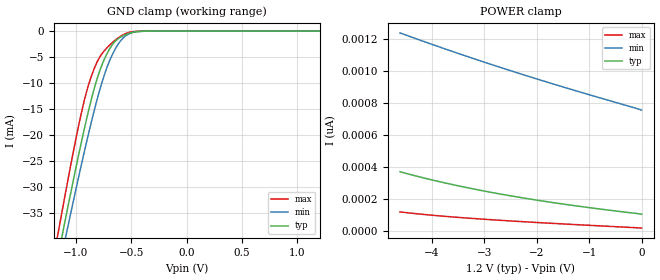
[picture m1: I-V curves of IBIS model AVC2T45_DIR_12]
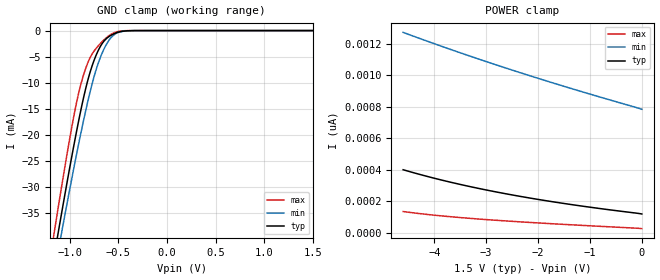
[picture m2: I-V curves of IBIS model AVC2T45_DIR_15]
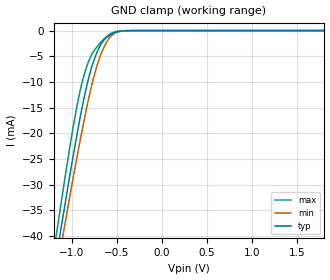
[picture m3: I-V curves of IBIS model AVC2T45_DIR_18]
| TEXAS INSTRUMENTS INCORPORATED
| Standard Linear and Logic Group
| IBIS Model of SN74AVC2T45
| DUAL-BIT DUAL-SUPPLY BUS TRANSCEIVER WITH CONFIGURABLE VOLTAGE
| TRANSLATION AND 3-STATE OUTPUTS
| This file contains package information for the following:
|  SOT 8-pin (DCT) package as [Component] AVC2T45_DCT
|  SOT 8-pin (DCU) package as [Component] AVC2T45_DCU
|  NanoStar WCSP 8-pin (YEP) package as [Component] AVC2T45_YEP
|  NanoFree WCSP 8-pin (YZP) package as [Component] AVC2T45_YZP
|  NanoFree WCSP 8-pin (YZT) package as [Component] AVC2T45_YZT
| This device can be powered at the following Vccs:
|  1.2 volt Vcc
|  1.5 volt Vcc
|  1.8 volt Vcc
|  2.5 volt Vcc
|  3.3 volt Vcc
| This file provides unique models under the [Model Selector] for each Vcc.
| For operation at a specific Vcc, select the appropriate model after each
| [Model Selector] keyword.
[IBIS Ver]   3.2
[Comment char]  |_char
[File Name]   sn74avc2t45.ibs
[File Rev]   1.2 | x_die
[Date]   February 22, 2005
[Source]   Data created from TI-SPICE simulations at TI-SLL.
[Notes]   The following is an IBIS list for the AVC2T45.
   Please contact sllibis@ti.com with questions and
   comments concerning SLL IBIS models.
   - 1.1 Release IBIS file on 04/23/04
   - 1.2 YEP, YZP, and YZT packages added. 02/22/05
   - Power clamp data deleted as there is no power-clamp diode.
   - Due to the fact that the Device is 4.6-V Input/Output
   tolarent, the I/O models has some Non-Monotonic Warnings.
   - End point warning due to AC and DC mismatch.
[Disclaimer] Property of Texas Instruments Incorporated.  Unauthorized
   reproduction and/or distribution is strictly prohibited.
   This product is protected under copyright law.
   Created  2004, (C) Copyright  2004, Texas Instruments
   Incorporated, All Rights Reserved
   UNLESS THERE IS A SIGNED, WRITTEN AGREEMENT TO THE
   CONTRARY, TEXAS INSTRUMENTS (TI) IS PROVIDING THE IBIS
   MODELS  AND WITHOUT ANY WARRANTY, EXPRESSED OR
   IMPLIED.  TI assumes no liability for:
   1) the accuracy of the IBIS models provided to your
   company;
   2) the proper functioning of these IBIS Models in your
   design or for any resulting applications; or
   3) infringement of patents, copyrights or intellectual
   property rights resulting from your use of these IBIS
   models.
   TI provides IBIS Models as a service to our customers.
   You and your company shall not distribute, sell or give
   these models to anyone else without prior written
   permission from TI.
   TI reserves the right to make changes to our products or
   to discontinue any semiconductor product or service
   without notice, and advises our customers to obtain the
   latest version of relevant information to verify, before
   placing orders, that the information being relied on is
   current.
   Please be aware that your receipt and use of the IBIS
   information provided shall serve as acceptance of these
   terms and conditions.  If you do not accept these terms,
   you should return or destroy the IBIS models and any
   other accompanying information immediately.
| Component AVC2T45_DCT 8-pin SOT
[Component]   AVC2T45_DCT
[Manufacturer]   Texas Instruments, Inc.
[Package]
|   typ   min   max
R_pkg   2.900e-02   2.800e-02   3.100e-02
L_pkg   1.796e-09   1.666e-09   1.924e-09
C_pkg   2.310e-13   2.210e-13   2.420e-13
[Pin]   signal_name   model_name   R_pin   L_pin   C_pin
1   VCCA   POWER   3.100e-02   1.894e-09   2.230e-13
2   A1   AVC2T45_IOA   2.800e-02   1.697e-09   2.370e-13
3   A2   AVC2T45_IOA   3.000e-02   1.722e-09   2.390e-13
4   GND   GND   3.000e-02   1.861e-09   2.210e-13
5   DIR   AVC2T45_DIR   2.800e-02   1.924e-09   2.280e-13
6   B2   AVC2T45_IOB   2.900e-02   1.736e-09   2.420e-13
7   B1   AVC2T45_IOB   2.800e-02   1.666e-09   2.360e-13
8   VCCB   POWER   3.000e-02   1.871e-09   2.220e-13
| Component AVC2T45_DCU 8-pin SOT
[Component]   AVC2T45_DCU
[Manufacturer]   Texas Instruments, Inc.
[Package]
|   typ   min   max
R_pkg   2.600e-02   2.300e-02   3.800e-02
L_pkg   1.394e-09   1.066e-09   2.046e-09
C_pkg   2.590e-13   2.150e-13   3.720e-13
[Pin]   signal_name   model_name   R_pin   L_pin   C_pin
1   VCCA   POWER   2.400e-02   1.520e-09   2.710e-13
2   A1   AVC2T45_IOA   2.300e-02   1.112e-09   2.180e-13
3   A2   AVC2T45_IOA   2.300e-02   1.070e-09   2.170e-13
4   GND   GND   2.700e-02   2.046e-09   3.720e-13
5   DIR   AVC2T45_DIR   2.700e-02   1.542e-09   2.730e-13
6   B2   AVC2T45_IOB   2.300e-02   1.100e-09   2.240e-13
7   B1   AVC2T45_IOB   2.300e-02   1.066e-09   2.150e-13
8   VCCB   POWER   3.800e-02   1.696e-09   2.800e-13
| Component AVC2T45_YEP 8-pin NanoStar WCSP
[Component]   AVC2T45_YEP
[Manufacturer]   Texas Instruments, Inc.
[Package]
|   typ   min   max
R_pkg   0.001   0.001   0.001
L_pkg   0.021nH   0.021nH   0.021nH
C_pkg   0.043pF   0.042pF   0.044pF
[Pin]   signal_name   model_name   R_pin   L_pin   C_pin
1   VCCA   POWER   0.046   2.861nH   0.321pF
2   A1   AVC2T45_IOA   0.037   2.437nH   0.286pF
3   A2   AVC2T45_IOA   0.034   2.419nH   0.286pF
4   GND   GND   0.043   2.784nH   0.321pF
5   DIR   AVC2T45_DIR   0.043   2.784nH   0.321pF
6   B2   AVC2T45_IOB   0.035   2.420nH   0.286pF
7   B1   AVC2T45_IOB   0.037   2.437nH   0.286pF
8   VCCB   POWER   0.046   2.860nH   0.321pF
| Component AVC2T45_YZP 8-pin NanoFree WCSP
[Component]   AVC2T45_YZP
[Manufacturer]   Texas Instruments, Inc.
[Package]
|   typ   min   max
R_pkg   0.001   0.001   0.001
L_pkg   0.021nH   0.021nH   0.021nH
C_pkg   0.043pF   0.042pF   0.044pF
[Pin]   signal_name   model_name   R_pin   L_pin   C_pin
1   VCCA   POWER   0.046   2.861nH   0.321pF
2   A1   AVC2T45_IOA   0.037   2.437nH   0.286pF
3   A2   AVC2T45_IOA   0.034   2.419nH   0.286pF
4   GND   GND   0.043   2.784nH   0.321pF
5   DIR   AVC2T45_DIR   0.043   2.784nH   0.321pF
6   B2   AVC2T45_IOB   0.035   2.420nH   0.286pF
7   B1   AVC2T45_IOB   0.037   2.437nH   0.286pF
8   VCCB   POWER   0.046   2.860nH   0.321pF
| Component AVC2T45_YZT 8-pin NanoFree WCSP
[Component]   AVC2T45_YZT
[Manufacturer]   Texas Instruments, Inc.
[Package]
|   typ   min   max
R_pkg   0.001   0.001   0.001
L_pkg   0.021nH   0.021nH   0.021nH
C_pkg   0.043pF   0.042pF   0.044pF
[Pin]   signal_name   model_name   R_pin   L_pin   C_pin
1   VCCA   POWER   0.046   2.861nH   0.321pF
2   A1   AVC2T45_IOA   0.037   2.437nH   0.286pF
3   A2   AVC2T45_IOA   0.034   2.419nH   0.286pF
4   GND   GND   0.043   2.784nH   0.321pF
5   DIR   AVC2T45_DIR   0.043   2.784nH   0.321pF
6   B2   AVC2T45_IOB   0.035   2.420nH   0.286pF
7   B1   AVC2T45_IOB   0.037   2.437nH   0.286pF
8   VCCB   POWER   0.046   2.860nH   0.321pF
| Model AVC2T45_DIR
[Model Selector]   AVC2T45_DIR
AVC2T45_DIR_12   1.2 volt Vcc
AVC2T45_DIR_15   1.5 volt Vcc
AVC2T45_DIR_18   1.8 volt Vcc
AVC2T45_DIR_25   2.5 volt Vcc
AVC2T45_DIR_33   3.3 volt Vcc
| Model AVC2T45_IOA
[Model Selector]   AVC2T45_IOA
AVC2T45_IOA_12   1.2 volt Vcc
AVC2T45_IOA_15   1.5 volt Vcc
AVC2T45_IOA_18   1.8 volt Vcc
AVC2T45_IOA_25   2.5 volt Vcc
AVC2T45_IOA_33   3.3 volt Vcc
| Model AVC2T45_IOB
[Model Selector]   AVC2T45_IOB
AVC2T45_IOB_12   1.2 volt Vcc
AVC2T45_IOB_15   1.5 volt Vcc
AVC2T45_IOB_18   1.8 volt Vcc
AVC2T45_IOB_25   2.5 volt Vcc
AVC2T45_IOB_33   3.3 volt Vcc
| Models and submodels in the file (15): AVC2T45_DIR_12 (Input), AVC2T45_DIR_15 (Input), AVC2T45_DIR_18 (Input), AVC2T45_DIR_25 (Input), AVC2T45_DIR_33 (Input), AVC2T45_IOA_12 (I/O), AVC2T45_IOA_15 (I/O), AVC2T45_IOA_18 (I/O), AVC2T45_IOA_25 (I/O), AVC2T45_IOA_33 (I/O), AVC2T45_IOB_12 (I/O), AVC2T45_IOB_15 (I/O), AVC2T45_IOB_18 (I/O), AVC2T45_IOB_25 (I/O), AVC2T45_IOB_33 (I/O)
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[Model]   AVC2T45_DIR_12
Model_type  Input
Vinl=0.42
Vinh=0.78
| variable   typ   min   max
C_comp   2.46pF   2.11pF   2.89pF
[Temperature Range]   40   100   -40
| Ambient temperature   25   85   -40
[Voltage range]   1.2   NA   NA
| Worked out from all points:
|   GND clamp passes 1 mA (typ) near -0.58 V on its own axis
[GND Clamp]
| AVC2T45_DIR_12
|   Voltage   I(typ)   I(min)   I(max)
-4.6V     -459.2mA   -437.9mA   -484.2mA
-1.165V   -43.78mA   -47mA      -39.35mA
-1.115V   -38.35mA   -41.89mA   -33.51mA
-1.09V    -35.67mA   -39.36mA   -30.63mA
-1.065V   -33.02mA   -36.85mA   -27.8mA
-945mV    -20.79mA   -25.16mA   -15.18mA
-840mV    -11.44mA   -15.71mA   -7.485mA
-710mV    -3.942mA   -6.433mA   -2.997mA
-630mV    -1.665mA   -2.889mA   -1.475mA
-555mV    -700.6uA   -964.8uA   -509.7uA
-385mV    -23.61uA   -32.06uA   -5.101uA
1.2V      106.8pA    765.6pA    17.5pA
[POWER Clamp]
| AVC2T45_DIR_12
|   Voltage   I(typ)   I(min)   I(max)
-4.6V     371.2pA    1.236nA    121.1pA
-4.14V    332.1pA    1.182nA    105.2pA
-3.655V   295.2pA    1.126nA    91.26pA
-3.14V    260.1pA    1.069nA    78.67pA
-2.6V     227.3pA    1.011nA    67.08pA
-2.035V   196.6pA    953.1pA    56.09pA
-1.44V    167.5pA    893.7pA    45.32pA
-75.56fV  106.8pA    755.3pA    20pA
[Model]   AVC2T45_DIR_15
Model_type  Input
Vinl=0.49
Vinh=1.04
| variable   typ   min   max
C_comp   2.41pF   2.01pF   2.90pF
[Temperature Range]   40   100   -40
| Ambient temperature   25   85   -40
[Voltage range]   1.5   1.4   1.6
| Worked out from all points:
|   GND clamp passes 1 mA (typ) near -0.58 V on its own axis
[GND Clamp]
| AVC2T45_DIR_15
|   Voltage   I(typ)   I(min)   I(max)
-4.6V     -459.2mA   -437.9mA   -484.2mA
-1.175V   -44.87mA   -48.03mA   -40.53mA
-1.145V   -41.6mA    -44.95mA   -37mA
-1.12V    -38.89mA   -42.4mA    -34.09mA
-1.095V   -36.21mA   -39.87mA   -31.21mA
-1.07V    -33.55mA   -37.35mA   -28.36mA
-945mV    -20.79mA   -25.16mA   -15.18mA
-840mV    -11.44mA   -15.71mA   -7.485mA
-775mV    -7.058mA   -10.58mA   -4.657mA
-700mV    -3.56mA    -5.9mA     -2.784mA
-545mV    -612.9uA   -811.6uA   -423.5uA
1.5V      118pA      793.8pA    21.88pA
[POWER Clamp]
| AVC2T45_DIR_15
|   Voltage   I(typ)   I(min)   I(max)
-4.6V     399.2pA    1.272nA    133.5pA
-4.14V    357.1pA    1.217nA    115.2pA
-3.655V   317.5pA    1.16nA     99.58pA
-3.145V   280.4pA    1.103nA    85.9pA
-2.6V     245.1pA    1.043nA    73.35pA
-2.04V    212.7pA    984.3pA    61.9pA
-1.445V   182pA      923.8pA    50.75pA
-75.56fV  118pA      783.3pA    24.65pA
[Model]   AVC2T45_DIR_18
Model_type  Input
Vinl=0.5775
Vinh=1.2675
| variable   typ   min   max
C_comp   2.36pF   1.92pF   2.90pF
[Temperature Range]   40   100   -40
| Ambient temperature   25   85   -40
[Voltage range]   1.8   1.65   1.95
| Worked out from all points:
|   GND clamp passes 1 mA (typ) near -0.58 V on its own axis
[GND Clamp]
| AVC2T45_DIR_18
|   Voltage   I(typ)   I(min)   I(max)
-4.6V     -459.2mA   -437.9mA   -484.2mA
-1.185V   -45.97mA   -49.06mA   -41.71mA
-1.155V   -42.69mA   -45.98mA   -38.17mA
-1.13V    -39.97mA   -43.42mA   -35.25mA
-1.105V   -37.28mA   -40.88mA   -32.35mA
-1.08V    -34.61mA   -38.36mA   -29.5mA
-950mV    -21.28mA   -25.63mA   -15.65mA
-840mV    -11.44mA   -15.71mA   -7.485mA
-765mV    -6.504mA   -9.869mA   -4.351mA
-695mV    -3.38mA    -5.644mA   -2.68mA
-540mV    -571.7uA   -743.1uA   -384.3uA
1.8V      129.6pA    822.2pA    26.26pA
